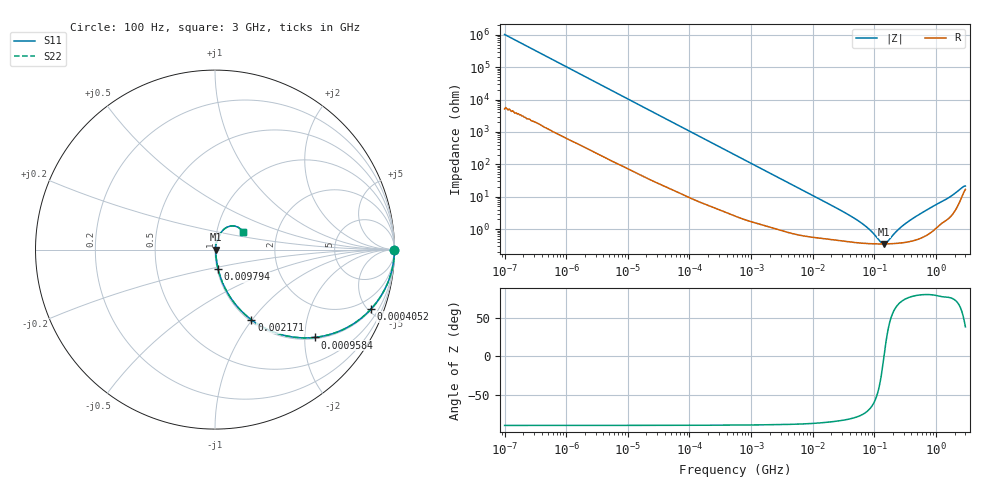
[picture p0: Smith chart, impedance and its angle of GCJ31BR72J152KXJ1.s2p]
!Murata Part Number: GCJ31BR72J152KXJ1
!These Parameters are Measured in Series Mode Connection
!Data Generated on Mar 13, 2026
!  o--ll--o
!Port1  Port2
!  o------o
!Operation Temp=25[degC], DC Bias Voltage=0[V]
!Freq. Start=100[Hz] Stop=3[GHz] 401[Steps]
# Hz S RI R 50
!Freq.(Hz) S11(Real) S11(Imag) S21(Real) S21(Imag) S12(Real) S12(Imag) S22(Real) S22(Imag)
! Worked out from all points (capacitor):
!   401 points, 100 Hz to 3 GHz, reference 50 ohm
!   read as one part in series: C = 1.55 nF near 109 Hz
!   lowest |Z| = 349 mohm at 141.2 MHz (marker M1)
!   series resonance near 143.2 MHz, so ESL is about 800 pH
!   S11 on the Smith chart (normalised r, x): 100 Hz: open; 405.2 kHz: 1.06, -5.26; 958.4 kHz: 1.03, -2.24; 2.171 MHz: 1.02, -0.99; 9.794 MHz: 1.01, -0.22; 3 GHz: 1.34, +0.27
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100  1 -9.75e-05  5e-07 9.75e-05  5e-07 9.75e-05  1 -9.75e-05
1788  1 -0.00172  1.4e-05 0.00172  1.4e-05 0.00172  1 -0.00172
31977  0.9988 -0.0304  0.00116 0.0304  0.00116 0.0304  0.9988 -0.0304
132342  0.9835 -0.1229  0.0165 0.1229  0.0165 0.1229  0.9835 -0.1229
405239  0.8706 -0.3297  0.1294 0.3297  0.1294 0.3297  0.8706 -0.3297
547723  0.7885 -0.4019  0.2115 0.4019  0.2115 0.4019  0.7885 -0.4019
958445  0.5546 -0.4893  0.4454 0.4893  0.4454 0.4893  0.5546 -0.4893
1411895  0.3691 -0.4735  0.6309 0.4735  0.6309 0.4735  0.3691 -0.4735
2171352  0.2033 -0.3915  0.7967 0.3915  0.7967 0.3915  0.2033 -0.3915
4141163  0.0705 -0.2418  0.9295 0.2418  0.9295 0.2418  0.0705 -0.2418
9794414  0.0176 -0.1087  0.9824 0.1087  0.9824 0.1087  0.0176 -0.1087
5.478864e7  0.00405 -0.0175  0.9959 0.0175  0.9959 0.0175  0.00405 -0.0175
8.070971e7  0.00364 -0.00956  0.9964 0.00956  0.9964 0.00956  0.00364 -0.00956
1.241234e8  0.00348 -0.00227  0.9965 0.00227  0.9965 0.00227  0.00348 -0.00227
1.412317e8  0.00347 -0.00022  0.9965 0.00022  0.9965 0.00022  0.00347 -0.00022
1.539281e8  0.00348 0.00115  0.9965 -0.00115  0.9965 -0.00115  0.00348 0.00115
1.751444e8  0.00352 0.00322  0.9965 -0.00322  0.9965 -0.00322  0.00352 0.00322
2.58007e8  0.00378 0.00991  0.9962 -0.00991  0.9962 -0.00991  0.00378 0.00991
3.967889e8  0.00456 0.0192  0.9954 -0.0192  0.9954 -0.0192  0.00456 0.0192
1.71441e9  0.0322 0.0928  0.9678 -0.0928  0.9678 -0.0928  0.0322 0.0928
2.525516e9  0.0958 0.1321  0.9042 -0.1321  0.9042 -0.1321  0.0958 0.1321
3e9  0.1548 0.0967  0.8452 -0.0967  0.8452 -0.0967  0.1548 0.0967
